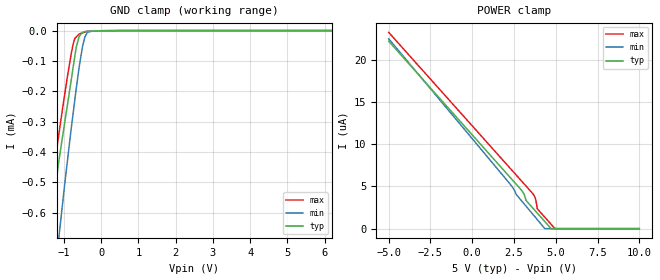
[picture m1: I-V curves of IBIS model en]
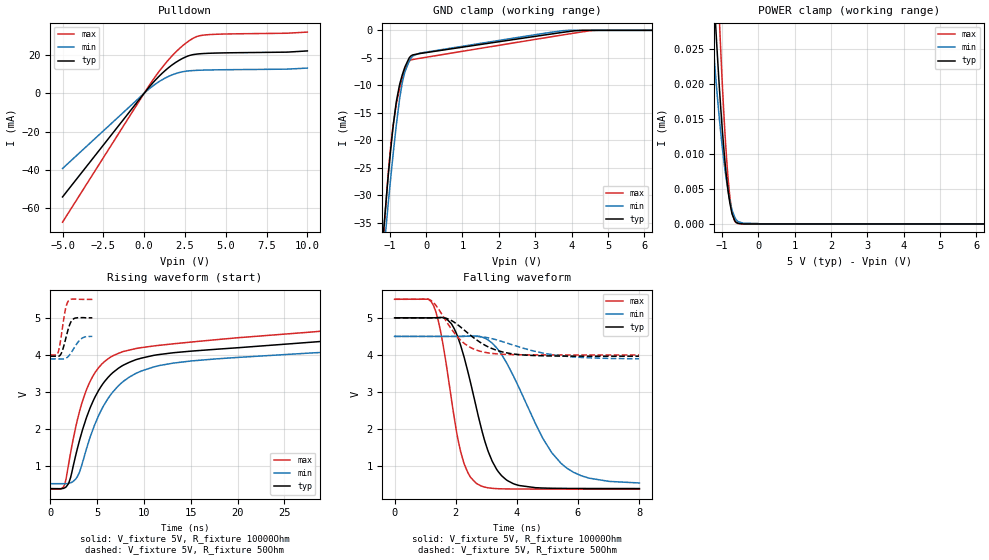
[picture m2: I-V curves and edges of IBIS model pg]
|Texas Instruments Incorporated
|4.5V to 18V Input, 3A Synchronous Step-Down DCAP2 Mode Converter with Eco-Mode
| Marketing part#   Digital Voltage Range   Package-type   #pins
| TPS54326PWP   4.5V - 18V   HTSSOP   14
| TPS54326PWPR   4.5V - 18V   HTSSOP   14
| TPS54326RGTR   4.5V - 18V   QFN   16
| TPS54326RGTT   4.5V - 18V   QFN   16
[IBIS Ver]   3.2
[File name]   tps54326.ibs
[File Rev]   1.0
[Date]   11/28/2012
[Source]
| Texas Instruments Incorporated.
| Analog-eLab Design Center, HPA
| 12500 TI Blvd
| Dallas, TX -75243
| e-mail: elab_scm_ibis@list.ti.com
[Notes]   Revision History:
| Rev 1.0: 11/28/2012
| - Initial version of the model
| - Model generated from simulations in TISPICE
| - Model matched to SPICE simulation
| - C_comp although listed in numerical order of value are
|   obtained from varying PVT conditions. For PVT conditions for
|   each specific value refer the buffer description under
|   respective [Model]. IBIS model user is responsible for using
|   appropriate C_comp to simulate for Signal Integrity.
| - Model names contains the model for 5.0V [4.5V and 5.5V].
|*   EXCEPTION:   *
|*   - For model en there will be a leakage current in the Power Clamp I-V   *
|*   table because of a resistor bank(R56) connected to the pad and GND   *
|*   clamp I-V table because of a transistor(MN8) connected on pad.   *
|*   - For model pg there will be a leakage current in the  GND  clamp I-V   *
|*   table because of a transistor(MP15) connected on pad.   *
[Disclaimer]
| This model is designed as an aid for customers of Texas Instruments.
| TI and its licensors and suppliers make no warranties, either expressed
| or implied, with respect to this  model, including the warranties of
| merchantability or fitness for a particular purpose. The model is
| provided solely on an "as is" basis. The entire risk as to its quality
| and performance is with the customer.
[Copyright]
(C) Copyright 2012 Texas Instruments Incorporated.All rights reserved.
|   TPS54326PWP
[Component]   TPS54326PWP
[Manufacturer]   TI
[Package]   |14 HTSSOP -  PWP  package
|   typ   min   max
R_pkg   0.04724   0.02283   0.06067
L_pkg   2.67598nH   2.08163nH   3.10261nH
C_pkg   0.49278pF   0.46464pF   0.53295pF
[Pin]  signal_name   model_name   R_pin   L_pin   C_pin
1   VO   term   0.05321   2.82938nH  0.46464pF
2   VFB   term   0.05760   2.93392nH  0.49532pF
3   VREG5   term   0.05391   2.80289nH  0.48706pF
4   SS   term   0.05023   2.67494nH  0.48171pF
5   GND   gnd   0.05070   2.69428nH  0.48296pF
6   PG   pg   0.05516   2.85521nH  0.48892pF
7   EN   en   0.06067   3.10261nH  0.47527pF
8   PGND1   gnd   0.02623   2.35843nH  0.50515pF
9   PGND2   gnd   0.02414   2.18930nH  0.52318pF
10   SW1   term   0.02428   2.12724nH  0.53295pF
11   SW2   term   0.02283   2.08163nH  0.51634pF
12   VBST   power   0.03814   2.25487nH  0.45756pF
13   VIN   power   0.01814   2.16819nH  0.55527pF
14   VCC   power   0.05275   2.81338nH  0.46814pF
|   TPS54326RGT
[Component]   TPS54326RGT
[Manufacturer]   TI
[Package]   |16 QFN   -  RGT package
|   typ   min   max
R_pkg   0.02522   0.01130   0.03161
L_pkg   0.83931nH   0.67483nH   0.93983nH
C_pkg   0.13370pF   0.10660pF   0.20160pF
[Pin]  signal_name   model_name   R_pin   L_pin   C_pin
1   VFB   term   0.03134   0.93433nH  0.10863pF
2   VREG5   term   0.02968   0.87793nH  0.11336pF
3   SS   term   0.02817   0.83016nH  0.11109pF
4   GND   gnd   0.03088   0.91947nH  0.10928pF
5   PG   pg   0.03083   0.91432nH  0.10660pF
6   EN   en   0.02977   0.87718nH  0.11199pF
7   PGND1   gnd   0.01064   0.61605nH  0.18625pF
8   PGND2   gnd   0.01522   0.63694nH  0.14579pF
9   SW1   term   0.01811   0.81924nH  0.17450pF
10   SW2   term   0.01130   0.67483nH  0.20160pF
11   SW3   term   0.01615   0.68594nH  0.16732pF
12   VBST   power   0.03024   0.88912nH  0.10879pF
13   VIN1   power   0.01622   0.68990nH  0.15293pF
14   VIN2   power   0.01036   0.59008nH  0.18165pF
15   VCC   power   0.03104   0.91941nH  0.11828pF
16   VO   term   0.03161   0.93983nH  0.10817pF
[Model] term
Model_type Terminator
C_comp   1.0e-20F  1.0e-20F  1.0e-20F
|   typ   min   max
[Voltage Range]   5.0V   4.5V   5.5V
[POWER Clamp Reference]   5.0V   4.5V   5.5V
[GND Clamp Reference]   0V   0V   0V
|Ambient Temperature   25   85   -40
|Junction Temperature
[Temperature Range]   27   125   -40
| Models and submodels in the file (3): en (Input), pg (Open_drain), term (Terminator)
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|   Model Selectors
|[Model Selector] en
|en   5.0V  digital input
|[Model Selector] pg
|pg   5.0V  digital Open_Drain
|[Model Selector] term
|term_5-0V   5.0V  nominal termination
|   en Model
[Model]   en
Model_type   Input
Vinl = 0.4
Vinh = 1.5
|   typ   min   max
|   (nom PVT)   (fast PVT)   (slow PVT)
|C_comp from frequency sweep method (F=700KHz)
|Average
|C_comp   3.972e-12   3.694e-12   4.121e-12
|C_comp from LC tank measurement(L=1nH)
|Average
|Resonant Frequency(Hz)   2.810e+09   2.910e+09   2.760e+09
C_comp   3.211e-12   2.994e-12   3.329e-12
| Where nom  PVT is Nominal Process, 5V, 27C
|   Fast PVT is Strong Process,  5.5V, -40C
|   Slow PVT is Weak Process,   4.5V, 125C
[Voltage Range]   5   4.5   5.5
|Ambient Temperature   25   85   -40
|Junction Temperature
[Temperature Range]   27   125   -40
[Power Clamp Reference]   5   4.5   5.5
[GND Clamp Reference]   0   0   0
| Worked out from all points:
|   GND clamp passes 1 mA (typ) near -1.75 V on its own axis
[GND Clamp]
|   Voltage   I(typ)   I(min)   I(max)
-5V       -4.582mA   -6.012mA   -4.201mA
-1.746V   -993.7uA   -1.389mA   -882.6uA
-1.375V   -643.6uA   -948.7uA   -545.2uA
-1.14V    -432uA     -685.2uA   -344.5uA
-1.028V   -342.4uA   -560.2uA   -249.2uA
-753.5mV  -121.4uA   -271.9uA   -44.91uA
-675mV    -58.29uA   -194.8uA   -21.76uA
-595mV    -20.13uA   -123.2uA   -11.62uA
-435mV    -3.053uA   -20.37uA   -4.597uA
-369mV    -2.683uA   -5.36uA    -2.25uA
153mV     -427.5nA   0A         -871.7nA
10V       0A         0A         0A
[POWER Clamp]
|   Voltage   I(typ)   I(min)   I(max)
-5V       22.22uA    22.5uA     23.26uA
2.268V    6.071uA    5.282uA    7.159uA
2.85V     4.777uA    3.545uA    5.869uA
3.085V    4.155uA    2.988uA    5.349uA
3.215V    3.356uA    2.68uA     5.061uA
3.624V    2.444uA    1.71uA     4.147uA
3.779V    2.101uA    1.345uA    3.562uA
3.894V    1.844uA    1.071uA    2.355uA
4.343V    846.5nA    0A         1.359uA
4.72V     0A         0A         520nA
4.95V     0A         0A         0A
10V       0A         0A         0A
|   pg Model
[Model]   pg
Model_type   Open_drain
Polarity   Non-Inverting
Vmeas = 2.5
Vref = 5
Cref = 2pF
Rref = 10000
|   typ   min   max
|   (nom PVT)   (fast PVT)   (slow PVT)
|C_comp from frequency sweep method (F=350KHz)
|C_comp   3.421e-12   3.058e-12   3.840e-12
|ON state : BUFFER OUTPUT TURNED LOW
|C_comp   3.421e-12   3.058e-12   3.840e-12
|OFF state: BUFFER IN HIGH IMPEDANCE
|C_comp   2.754e-12   2.565e-12   2.950e-12
|C_comp from LC tank measurement(L=1nH)
|Resonant Frequency(Hz)   4.120e+09   4.170e+09   4.020e+09
C_comp   1.494e-12   1.458e-12   1.569e-12
|ON state : BUFFER OUTPUT TURNED LOW
|Resonant Frequency(Hz)   4.120e+09   4.170e+09   4.020e+09
|C_comp   1.494e-12   1.458e-12   1.569e-12
|OFF state: BUFFER IN HIGH IMPEDANCE
|Resonant Frequency(Hz)   4.140e+09   4.210e+09   4.040e+09
|C_comp   1.479e-12   1.431e-12   1.553e-12
| Where nom  PVT is Nominal Process, 5V, 27C
|   Fast PVT is Strong Process,  5.5V, -40C
|   Slow PVT is Weak Process,   4.5V, 125C
[Voltage Range]   5   4.5   5.5
|Ambient Temperature   25   85   -40
|Junction Temperature
[Temperature Range]   27   125   -40
[Pullup Reference]   5   4.5   5.5
[Pulldown Reference]   0   0   0
[Power Clamp Reference]   5   4.5   5.5
[GND Clamp Reference]   0   0   0
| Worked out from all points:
|   slope of the pulldown table from 0 to 0.75 V, typ, clamps not added: 101 ohm
|   falling waveform, V_fixture 5V, R_fixture 10000Ohm: 20-80 % time 878ps typ, 1.46ns min, 616ps max; typ from 5 V to 0.399 V
|   rising waveform, V_fixture 5V, R_fixture 10000Ohm: 20-80 % time 11.2ns typ, 7.78ns min, 18.4ns max; typ from 0.397 V to 5 V
|   falling waveform, V_fixture 5V, R_fixture 50Ohm: 20-80 % time 1.09ns typ, 1.64ns min, 831ps max; typ from 5 V to 3.97 V
|   rising waveform, V_fixture 5V, R_fixture 50Ohm: 20-80 % time 677ps typ, 964ps min, 555ps max; typ from 3.97 V to 5 V
[Pulldown]
|   Voltage   I(typ)   I(min)   I(max)
-5V       -54.02mA   -39.2mA    -67.19mA
456mV     4.698mA    3.309mA    5.931mA
984mV     9.462mA    6.456mA    12.15mA
1.523V    13.54mA    8.917mA    17.75mA
2.167V    17.32mA    10.87mA    23.36mA
2.595V    19.13mA    11.57mA    26.39mA
3.235V    20.45mA    11.97mA    29.61mA
3.795V    20.8mA     12.13mA    30.47mA
8.684V    21.45mA    12.59mA    31.31mA
10V       22.09mA    13.14mA    31.91mA
[GND Clamp]
|   Voltage   I(typ)   I(min)   I(max)
-5V       -450.5mA   -412.3mA   -505.3mA
-1.25V    -43.04mA   -46.94mA   -44.8mA
-1.046V   -26.93mA   -31.95mA   -26.49mA
-920mV    -18.43mA   -23.54mA   -18.12mA
-809mV    -12.69mA   -16.81mA   -13.17mA
-720.5mV  -9.723mA   -12.23mA   -10.4mA
-610mV    -7.23mA    -8.259mA   -7.752mA
-462.5mV  -5.008mA   -5.603mA   -5.59mA
-363.5mV  -4.466mA   -4.668mA   -5.298mA
3.878V    -258.6uA   -10.55uA   -709.9uA
4.73V     0A         0A         -33.01nA
10V       0A         0A         0A
[POWER Clamp]
|   Voltage   I(typ)   I(min)   I(max)
-5V       4.347mA    3.983mA    5.986mA
-1.843V   118uA      81.31uA    199.5uA
-1.25V    36.69uA    26.6uA     55.53uA
-1.157V   27.47uA    20.43uA    41.5uA
-1.065V   19.49uA    15.05uA    29.27uA
-1.036V   17.18uA    13.48uA    25.71uA
-915mV    9.145uA    7.905uA    13.3uA
-806mV    4uA        4.119uA    5.385uA
-710mV    1.351uA    1.887uA    1.495uA
-644mV    491.4nA    960.6nA    424.7nA
-549.5mV  82.61nA    325.9nA    46.68nA
10V       0A         0A         0A
[Ramp]
R_load = 10000
|   typ   min   max
dV/dt_r   2.73165/9.74669e-09   2.35737/7.33362e-09   3.03511/1.62613e-08
dV/dt_f   2.7619/8.93161e-10   2.38148/1.50491e-09   3.0712/6.16517e-10
[Falling Waveform]
V_fixture = 5V
V_fixture_min = 4.5V
V_fixture_max = 5.5V
R_fixture = 10000Ohm
|   Time   V(typ)   V(min)   V(max)
0s        5V         4.5V       5.5V
1.275ns   5.001V     4.499V     5.327V
1.535ns   5.011V     4.499V     4.505V
2.15ns    4.284V     4.5V       1.432V
2.655ns   2.65V      4.507V     552.7mV
3.195ns   1.133V     4.316V     405.6mV
3.875ns   534.5mV    3.453V     388.2mV
4.85ns    413.8mV    1.751V     385.4mV
5.455ns   404.5mV    1.072V     384.7mV
8.01ns    399.4mV    550.5mV    383.2mV
[Rising Waveform]
V_fixture = 5V
V_fixture_min = 4.5V
V_fixture_max = 5.5V
R_fixture = 10000Ohm
|   Time   V(typ)   V(min)   V(max)
0s        396.8mV    530.1mV    381.3mV
1.38ns    401.3mV    529.6mV    433.2mV
1.96ns    536.7mV    537.2mV    1.061V
3.39ns    1.935V     1.053V     2.714V
5.13ns    3.03V      2.346V     3.646V
7.67ns    3.706V     3.259V     4.081V
11.42ns   4.003V     3.7V       4.253V
34.71ns   4.475V     4.142V     4.768V
70.03ns   4.852V     4.389V     5.308V
167ns     4.998V     4.497V     5.498V
[Falling Waveform]
V_fixture = 5V
V_fixture_min = 4.5V
V_fixture_max = 5.5V
R_fixture = 50Ohm
|   Time   V(typ)   V(min)   V(max)
0s        5V         4.5V       5.5V
1.175ns   5V         4.5V       5.476V
1.35ns    5.002V     4.5V       5.337V
1.705ns   4.982V     4.5V       4.888V
2.145ns   4.761V     4.5V       4.41V
2.47ns    4.539V     4.503V     4.206V
2.87ns    4.303V     4.488V     4.085V
3.78ns    4.039V     4.292V     4.011V
5.245ns   3.971V     3.997V     4V
7.995ns   3.966V     3.897V     3.999V
[Rising Waveform]
V_fixture = 5V
V_fixture_min = 4.5V
V_fixture_max = 5.5V
R_fixture = 50Ohm
|   Time   V(typ)   V(min)   V(max)
0s        3.966V     3.893V     3.999V
650ps     3.966V     3.893V     3.999V
835ps     3.963V     3.893V     4.066V
1.205ns   4.059V     3.891V     4.566V
1.595ns   4.385V     3.901V     5.199V
1.94ns    4.714V     3.965V     5.458V
2.21ns    4.893V     4.054V     5.499V
2.52ns    4.979V     4.178V     5.506V
3.4ns     5.005V     4.453V     5.498V
4.49ns    5V         4.499V     5.497V
